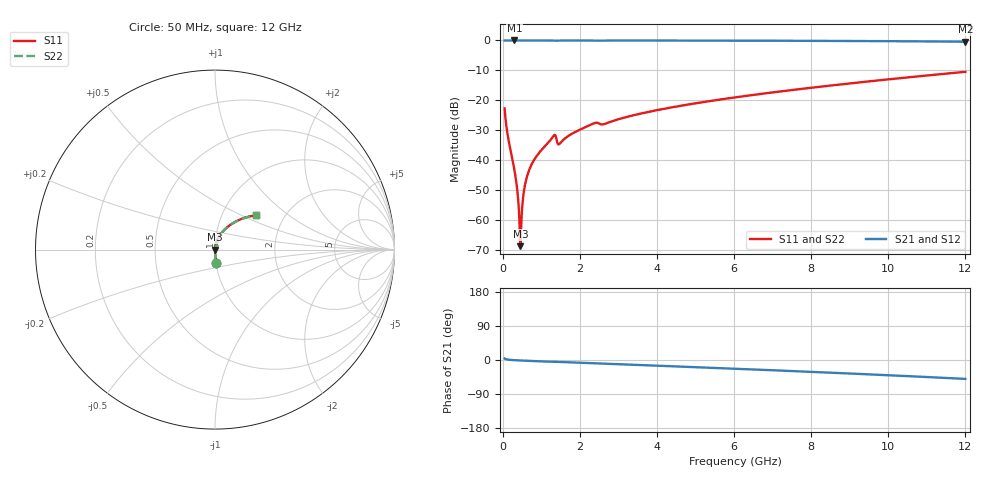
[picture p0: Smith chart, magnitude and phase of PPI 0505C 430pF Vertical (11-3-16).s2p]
# GHz S MA R 50
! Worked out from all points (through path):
!   1601 points, 50 MHz to 12 GHz, reference 50 ohm
!   highest |S21| = 0.00 dB at 303.9 MHz (marker M1); lowest = -0.4 dB at 12 GHz (marker M2)
!   group delay of S21, straight-line fit = 11.5 ps
!   lowest |S11| = -68.8 dB at 460.8 MHz (marker M3), VSWR 1.00, Z = 50 + j0.00683 ohm
!   |S11| at or under -10 dB: start of sweep to end of sweep
!   |S22| runs from -68.8 to -10.5 dB; largest |S21 - S12| = 0
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0.05  0.07288 -85.8  0.9972 4.0  0.9972 4.0  0.07288 -85.8
0.1545625  0.02121 -88.5  0.9995 0.8  0.9995 0.8  0.02121 -88.5
0.3039375  0.006845 -87.9  0.9996 -0.5  0.9996 -0.5  0.006845 -87.9
0.3636875  0.003801 -85.9  0.9996 -0.8  0.9996 -0.8  0.003801 -85.9
0.4234375  0.00134 -76.2  0.9996 -1.1  0.9996 -1.1  0.00134 -76.2
0.4607812  0.0003628 10.8  0.9996 -1.3  0.9996 -1.3  0.0003628 10.8
0.498125  0.001392 73.3  0.9996 -1.5  0.9996 -1.5  0.001392 73.3
0.557875  0.003231 81.5  0.9996 -1.7  0.9996 -1.7  0.003231 81.5
0.617625  0.004945 83.4  0.9996 -2.0  0.9996 -2.0  0.004945 83.4
0.7221875  0.007722 84.4  0.9995 -2.5  0.9995 -2.5  0.007722 84.4
0.8640937  0.01124 84.5  0.9994 -3.1  0.9994 -3.1  0.01124 84.5
1.312219  0.02506 75.6  0.9955 -5.1  0.9955 -5.1  0.02506 75.6
1.476531  0.0187 72.8  0.9958 -5.2  0.9958 -5.2  0.0187 72.8
1.715531  0.0256 81.2  0.9984 -6.2  0.9984 -6.2  0.0256 81.2
2.044156  0.03314 80.5  0.9982 -7.6  0.9982 -7.6  0.03314 80.5
2.387719  0.04169 75.2  0.9948 -9.0  0.9948 -9.0  0.04169 75.2
2.626719  0.03983 74.4  0.9949 -9.6  0.9949 -9.6  0.03983 74.4
4.038312  0.06901 74.0  0.9963 -15.2  0.9963 -15.2  0.06901 74.0
6.025  0.1116 66.4  0.9923 -23.0  0.9923 -23.0  0.1116 66.4
8.019156  0.1623 58.2  0.9849 -31.3  0.9849 -31.3  0.1623 58.2
10.01331  0.224 49.4  0.9724 -40.2  0.9724 -40.2  0.224 49.4
12  0.2989 39.8  0.9517 -49.9  0.9517 -49.9  0.2989 39.8
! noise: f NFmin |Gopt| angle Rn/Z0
0.05  0.0003042  0.8298  0.2125  0.0003765
1.372  0.01177  0.8763  3.809  0.02052
2.701  0.00889  0.707  7.366  0.00594
4.031  0.006764  0.4974  10.17  0.002304
5.36  0.00808  0.4576  13.03  0.002472
6.682  0.009515  0.437  15.73  0.002752
8.012  0.01103  0.426  18.32  0.003088
9.341  0.01264  0.4223  20.8  0.003484
10.67  0.01437  0.4246  23.22  0.003957
12  0.01627  0.4323  25.61  0.004531
